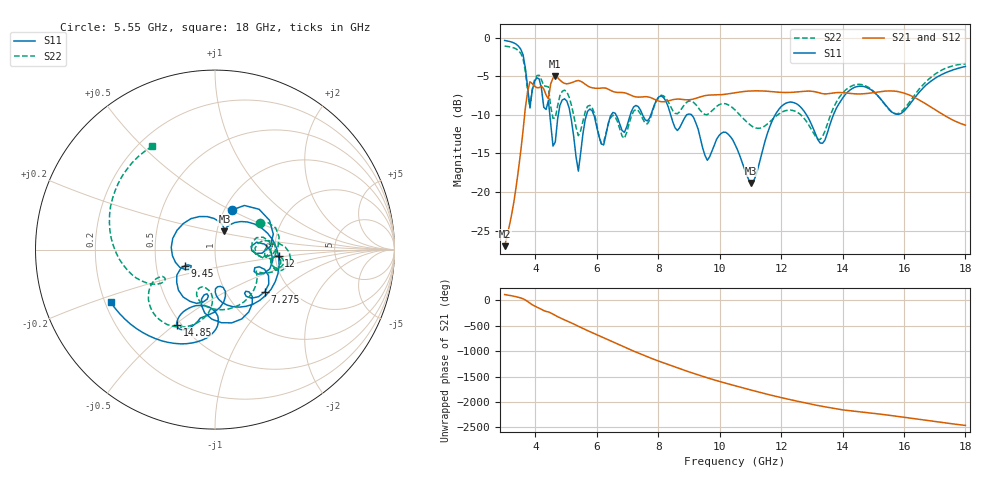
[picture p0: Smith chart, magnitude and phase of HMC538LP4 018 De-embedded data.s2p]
! Chelmsford, MA 01824
! http://www.hittite.com
! Tel: 978-250-3343
! Fax: 978-250-3373
! Device  :  HMC538LP4
! Description:  600 Analog Phase Shifter
! Frequency  :  6.0 GHz - 15.0 GHz
! Package  :  LP4  - 4x4 mm Quad Flatpack No-Lead (QFN) Plastic Package: 24 pin
! Ports  :  2 RF, 1 DC
!  Pin  3  = Rfin  = Port 1
!  Pin  16  = Rfout = Port 2
!  pin  21  = vCTL
! Voltages:  VCTL  = 0 to 5.0 Volts
! Currents :  Vb(V)  Vd(V)  Ib(mA)  Id(mA)
!  0.00  1.80  0.000000	0.479475
! Data:  The device was measured on evaluation board 111296-1.
!  Data was collected using a calibrated network analyzer.
!  The evaluation circuit board was modeled and simulated.This was use
!  to removed the evaluation board circuit from the measured data.
!  The reference plane is the center of the package pin.
! Misc:  Lot #
!Date Measured:  03 - 11 -2009
! Date:  03 - 17 -2009
! Note:
!  Hittite Microwave supplies this data as a sample of measured data at the
!  package pin for this package product.  Your particular data for this product
!  may vary.
!  Data was taken at 25 degrees C.
!  Hittite Microwave reserves the right to change this data at anytime.
# MHz S MA R 50
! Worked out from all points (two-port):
!   201 points, 3 GHz to 18 GHz, reference 50 ohm
!   highest |S21| = -5.03 dB at 4.65 GHz (marker M1); lowest = -27.0 dB at 3 GHz (marker M2)
!   |S21| within 3 dB of the highest: 3.713 GHz to 7.899 GHz (4.186 GHz wide, 72.1 % of centre); 9.056 GHz to 16.47 GHz (7.417 GHz wide, 58.1 % of centre)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
!   lowest |S11| = -18.8 dB at 11.03 GHz (marker M3), VSWR 1.26, Z = 54.3 + j11.2 ohm
!   |S11| at or under -10 dB: 5.902 GHz to 6.473 GHz (570.8 MHz wide, 9.22 % of centre); 9.086 GHz to 11.81 GHz (2.725 GHz wide, 26.1 % of centre); 12.83 GHz to 13.71 GHz (878.1 MHz wide, 6.62 % of centre)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
!   |S22| runs from -13.8 to -1.1 dB; largest |S21 - S12| = 0.0013
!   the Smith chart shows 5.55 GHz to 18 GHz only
!   S11 on the Smith chart (normalised r, x): 5.55 GHz: 1.08, +0.51; 7.275 GHz: 1.51, -0.81; 9.45 GHz: 0.70, -0.13; 12 GHz: 2.09, -0.18; 14.85 GHz: 0.47, -0.51; 18 GHz: 0.22, -0.23
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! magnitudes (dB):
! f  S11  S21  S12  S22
! 3 GHz  -0.4  -27.0  -27.0  -1.1
! 3.6 GHz  -2.2  -12.1  -12.0  -2.7
! 3.825 GHz  -9.0  -5.7  -5.7  -9.1
! 4.125 GHz  -5.4  -6.5  -6.5  -4.9
! 4.65 GHz  -13.5  -5.0  -5.0  -10.4
! 4.95 GHz  -7.9  -5.9  -5.9  -6.8
! 5.4 GHz  -17.3  -5.5  -5.6  -12.7
! 5.55 GHz  -12.4  -5.8  -5.8  -10.8
! 5.775 GHz  -9.2  -6.4  -6.4  -8.8
! 6.15 GHz  -13.7  -6.5  -6.5  -13.8
! 7.275 GHz  -8.8  -7.7  -7.7  -9.3
! 8.025 GHz  -7.7  -8.2  -8.2  -7.7
! 9.45 GHz  -14.3  -7.6  -7.6  -9.8
! 10.5 GHz  -13.8  -7.1  -7.1  -9.4
! 11.03 GHz  -18.8  -6.9  -6.9  -11.4
! 12 GHz  -9.0  -7.1  -7.1  -9.7
! 13.05 GHz  -11.8  -7.0  -7.0  -12.3
! 13.35 GHz  -13.7  -7.3  -7.3  -12.8
! 14.03 GHz  -7.7  -7.1  -7.2  -7.1
! 14.85 GHz  -6.6  -7.2  -7.2  -6.5
! 15.53 GHz  -9.3  -6.9  -6.9  -9.4
! 18 GHz  -3.7  -11.3  -11.3  -3.4
